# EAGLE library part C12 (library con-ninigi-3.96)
NINIGI
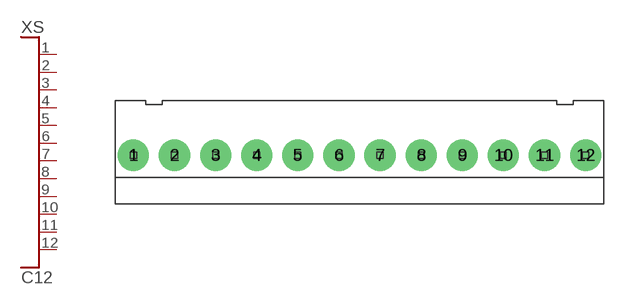
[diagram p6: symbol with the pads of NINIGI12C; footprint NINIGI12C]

Designator prefix XS

## C12  [NINIGI12C]
1  P$1
2  P$2
3  P$3
4  P$4
5  P$5
6  P$6
7  P$7
8  P$8
9  P$9
10  P$10
11  P$11
12  P$12

## Footprint NINIGI12C (pad centres in mm)
drill 1.6 pad 3: 1 -21.78,0; 2 -17.82,0; 3 -13.86,0; 4 -9.9,0; 5 -5.94,0; 6 -1.98,0; 7 1.98,0; 8 5.94,0; 9 9.9,0; 10 13.86,0; 11 17.82,0; 12 21.78,0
